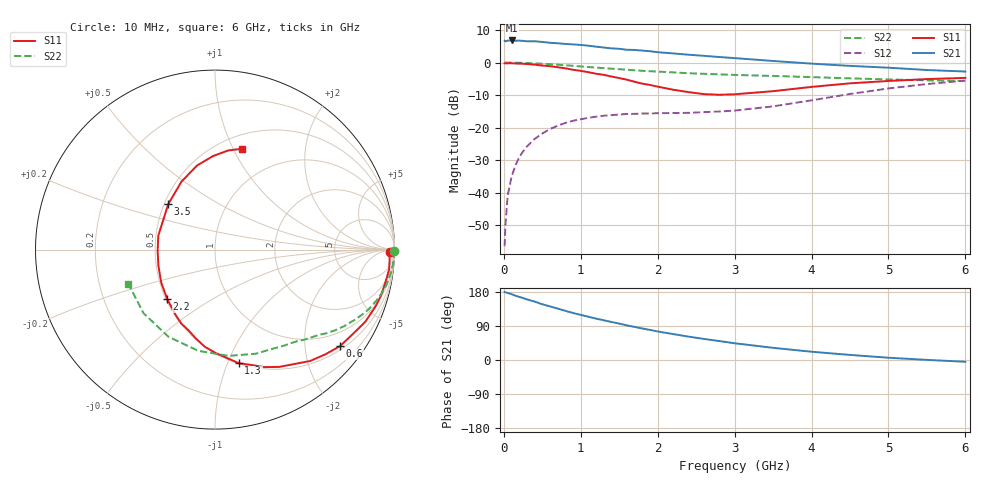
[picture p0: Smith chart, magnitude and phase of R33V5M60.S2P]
! SIEMENS Small Signal Semiconductors
! BFR181
! Si NPN RF Bipolar Junction Transistor in SOT23
! VCE = 3.5 V  IC = 0.6 mA
! Common Emitter S-Parameters:  May  1996
# GHz  S  MA  R  50
!  f  S11  S21  S12  S22
! GHz  MAG  ANG  MAG  ANG  MAG  ANG  MAG  ANG
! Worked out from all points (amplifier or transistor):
!   36 points, 10 MHz to 6 GHz, reference 50 ohm
!   highest |S21| = 6.8 dB at 100 MHz (marker M1)
!   |S21| within 3 dB of that: start of sweep to 1.741 GHz
!   unconditionally stable (mu >= 1): 2.275 GHz to 3.871 GHz
!   at 250 MHz: K = 0.13, MSG = 17.0 dB, |S12| = -27.3 dB
!   at 1.4 GHz: K = 0.65, MSG = 10.3 dB, |S12| = -16.2 dB
!   at 6 GHz: K = 0.91, MSG = 1.4 dB, |S12| = -5.5 dB
!   S11 on the Smith chart (normalised r, x): 10 MHz: 61, -34; 600 MHz: 0.59, -2.82; 1.3 GHz: 0.50, -1.10; 2.2 GHz: 0.51, -0.33; 3.5 GHz: 0.53, +0.31; 6 GHz: 0.64, +1.08
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0.01  0.9755 -0.8  2.162 179.7  0.0015 91.7  0.9998 -0.4
0.02  0.9709 -1.0  2.117 178.6  0.0031 88.8  0.9997 -0.7
0.05  0.9747 -3.2  2.177 177.0  0.009 88.8  0.9985 -1.5
0.1  0.9762 -6.5  2.188 173.8  0.0175 84.8  0.9969 -3.0
0.15  0.9699 -9.4  2.161 169.7  0.0261 82.8  0.9949 -4.6
0.25  0.9586 -15.9  2.154 163.4  0.0432 78.4  0.9886 -7.6
0.4  0.9292 -25.6  2.126 154.1  0.0669 72.8  0.9735 -11.9
0.5  0.8993 -31.8  2.079 147.1  0.0811 68.4  0.9591 -14.8
0.6  0.88 -37.7  2.016 141.5  0.095 64.9  0.9443 -17.4
0.9  0.7749 -55.4  1.902 124.0  0.1274 54.6  0.8915 -24.4
1.1  0.7102 -67.2  1.817 114.1  0.1413 49.0  0.854 -28.5
1.3  0.6463 -78.2  1.705 104.8  0.1522 44.3  0.8209 -32.2
1.6  0.5448 -95.9  1.574 91.3  0.1619 39.3  0.7775 -36.8
1.8  0.4733 -108.2  1.529 83.2  0.1647 37.9  0.7477 -39.5
2.2  0.3825 -134.2  1.383 68.5  0.1673 36.6  0.7063 -45.3
2.4  0.3512 -148.6  1.321 61.7  0.1685 37.9  0.6855 -48.1
2.8  0.3196 -178.7  1.217 50.0  0.1766 41.4  0.6588 -54.3
3.5  0.363 135.9  1.058 32.1  0.2119 48.8  0.623 -68.6
4.5  0.4793 102.0  0.889 13.4  0.3289 49.4  0.5715 -99.4
5  0.5213 91.2  0.834 6.0  0.3999 44.1  0.5506 -118.1
5.5  0.5573 82.4  0.768 0.3  0.4676 36.8  0.533 -138.3
6  0.5816 75.0  0.728 -4.7  0.5281 28.2  0.5194 -158.4
